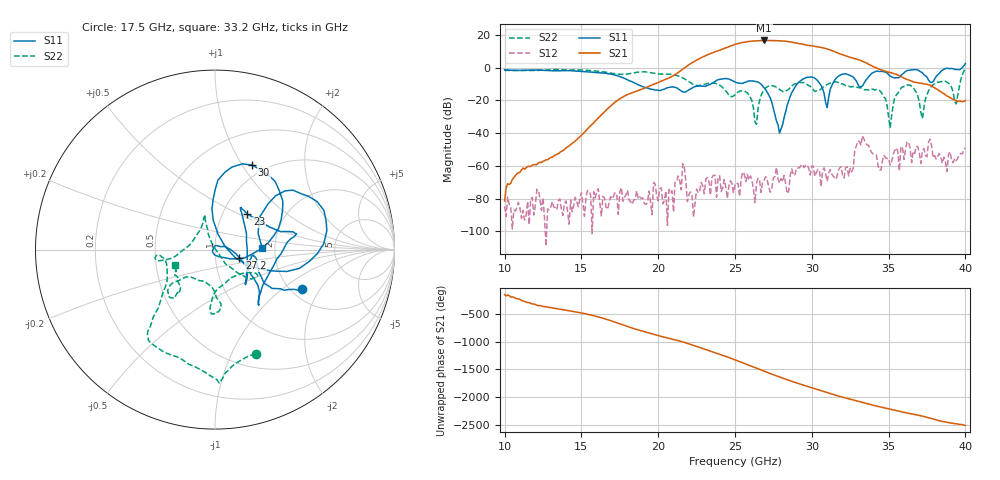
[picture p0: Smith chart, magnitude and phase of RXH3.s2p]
!Keysight Technologies,M9808A,MY58100618,A.14.70.03
!Date: Monday, February 27, 2023 13:24:43
!Correction: S11(Cdelta 2-Port  )
!S21(Cdelta 2-Port  )
!S12(Cdelta 2-Port  )
!S22(Cdelta 2-Port  )
!S2P File: Measurements: S11, S21, S12, S22:
# Hz S  RI  R 50
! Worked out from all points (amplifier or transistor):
!   301 points, 10 GHz to 40 GHz, reference 50 ohm
!   highest |S21| = 16.6 dB at 26.9 GHz (marker M1)
!   |S21| within 3 dB of that: 24.82 GHz to 29.74 GHz (4.923 GHz wide, 18 % of centre)
!   unconditionally stable (mu >= 1): start of sweep to 39.73 GHz
!   at 15 GHz: K = 46420.79, MAG = -32.2 dB, |S12| = -76.3 dB
!   at 25 GHz: K = 311.10, MAG = 14.9 dB, |S12| = -71.5 dB
!   at 40 GHz: K = -12.67, MSG = 14.4 dB, |S12| = -48.9 dB
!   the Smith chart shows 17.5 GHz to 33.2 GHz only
!   S11 on the Smith chart (normalised r, x): 17.5 GHz: 2.26, -1.40; 23 GHz: 1.30, +0.56; 27.2 GHz: 1.31, -0.12; 30 GHz: 0.86, +1.11; 33.2 GHz: 1.71, +0.03
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1e10  0.0325 0.8592  -7.36e-05 -4.04e-05  4.41e-05 -3.76e-05  0.7485 0.3349
1.5e10  0.729 0.2224  -0.00475 -0.00714  -4.26e-05 0.000146  0.6116 -0.5802
1.75e10  0.4824 -0.2222  0.0844 0.0733  0.000116 -0.00011  0.2274 -0.5835
2e10  0.1973 -0.0549  -0.3469 -0.0553  -7.58e-05 -4.08e-05  -0.1774 -0.6161
2.19e10  0.1756 0.0855  0.7477 0.8581  5.98e-06 8.06e-05  -0.2978 -0.2651
2.3e10  0.1797 0.1977  1.303 -1.787  0.000137 3.43e-05  -0.3044 -0.0329
2.39e10  0.4152 0.1004  -2.476 -2.134  0.000255 -0.000376  -0.2998 -0.061
2.45e10  0.4502 0.0845  -4.003 1.131  -6.15e-05 8.12e-05  -0.1705 0.00298
2.5e10  0.3675 -0.0241  -1.957 4.714  -0.000166 -0.000208  -0.0744 0.1279
2.55e10  0.2663 -0.1979  3.13 4.948  -0.000212 -0.000616  -0.0516 0.1928
2.6e10  0.2456 -0.3085  6.296 0.3041  -0.000486 -9.31e-05  -0.042 0.116
2.69e10  0.1989 -0.1378  -0.5884 -6.711  -0.000309 0.000202  0.1496 -0.1416
2.72e10  0.1361 -0.0454  -4.004 -5.4  -4.64e-05 -0.000221  0.2231 -0.1573
2.78e10  -0.00644 0.0166  -6.512 0.9249  -0.000235 -0.000309  0.1922 -0.127
2.85e10  0.083 -0.0512  -1.351 6.049  -1.7e-05 0.000173  0.0161 -0.2162
2.93e10  0.3685 0.1673  4.656 2.566  -0.00103 0.000105  0.00182 -0.3486
3e10  0.2071 0.4712  3.936 -2.465  -0.000461 0.000886  0.000876 -0.2392
3.07e10  -0.0171 0.2285  -0.2789 -4.028  8.09e-05 0.000661  -0.1878 -0.1641
3.14e10  0.3322 -0.1198  -2.895 -1.331  -0.000168 0.000452  -0.2603 -0.2431
3.32e10  0.2626 0.00944  0.5877 1.524  -0.000962 -0.00407  -0.2253 -0.0861
3.5e10  0.5958 0.1615  0.4576 -0.5607  -0.000683 0.00155  -0.0321 -0.00303
4e10  1.211 -0.5545  0.0988 0.0146  0.00273 -0.00233  0.4498 -0.8869
